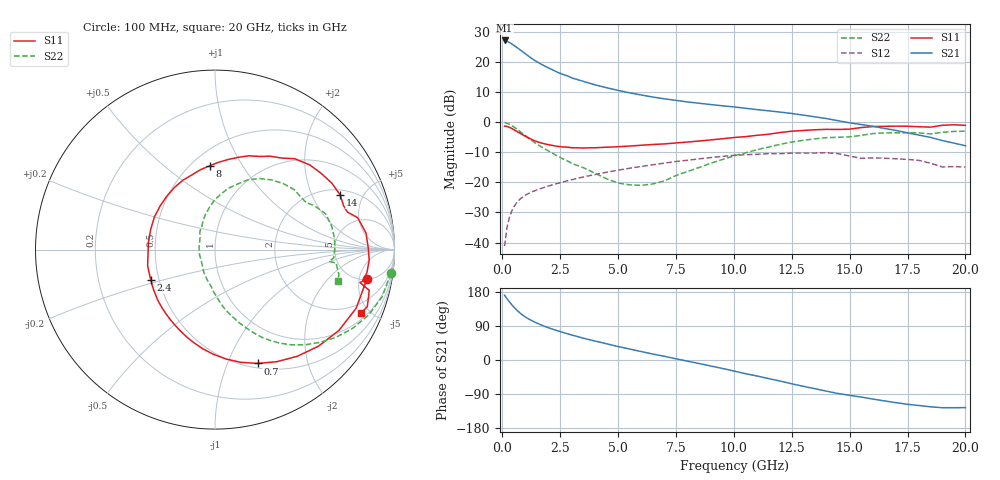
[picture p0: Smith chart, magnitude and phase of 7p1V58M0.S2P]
! Infineon Technologies  Discrete & RF Semiconductors
! bfp620
! VCE =  1.5 V,  IC =  8.0 mA
! Common Emitter S-Parameters:  Sep 2002
# GHz  S  MA  R  50
!  f  S11  S21  S12  S22
! GHz  MAG  ANG  MAG  ANG  MAG  ANG  MAG  ANG
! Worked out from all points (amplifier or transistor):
!   59 points, 100 MHz to 20 GHz, reference 50 ohm
!   highest |S21| = 27.2 dB at 100 MHz (marker M1)
!   |S21| within 3 dB of that: start of sweep to 747.6 MHz
!   unconditionally stable (mu >= 1): 4.357 GHz to 10.87 GHz; 17.09 GHz to end of sweep
!   at 1 GHz: K = 0.43, MSG = 23.5 dB, |S12| = -24.2 dB
!   at 5.5 GHz: K = 1.04, MAG = 11.2 dB, |S12| = -15.3 dB
!   at 20 GHz: K = 1.38, MAG = -0.1 dB, |S12| = -14.9 dB
!   S11 on the Smith chart (normalised r, x): 100 MHz: 5.18, -6.52; 700 MHz: 0.55, -1.29; 2.4 GHz: 0.45, -0.18; 8 GHz: 0.61, +0.73; 14 GHz: 2.28, +3.30; 20 GHz: 1.33, -4.40
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0.1  0.8621 -10.8  22.84 170.9  0.0087 84.8  0.9881 -7.6
0.2  0.8518 -22.5  22.2 162.0  0.0176 79.3  0.9676 -15.8
0.3  0.8245 -33.1  21.25 154.0  0.0256 73.8  0.9302 -23.1
0.4  0.7888 -43.0  20.13 146.5  0.0328 69.0  0.8835 -29.8
0.5  0.7505 -52.4  18.96 139.6  0.0392 64.8  0.8328 -35.9
0.6  0.7129 -61.2  17.81 133.3  0.0449 61.1  0.7813 -41.4
0.7  0.6772 -69.5  16.69 127.5  0.0498 58.0  0.731 -46.5
0.9  0.6124 -84.3  14.61 117.6  0.058 52.9  0.6375 -55.0
1  0.5832 -90.9  13.67 113.4  0.0614 50.9  0.5951 -58.5
1.2  0.532 -102.8  12 106.2  0.0673 47.7  0.5202 -64.4
1.4  0.4913 -113.4  10.65 100.1  0.0725 45.4  0.4583 -69.2
1.9  0.4309 -135.8  8.347 87.2  0.0846 41.6  0.3487 -79.1
2.4  0.3961 -154.5  6.728 76.9  0.0964 38.6  0.2717 -87.0
3.5  0.3734 173.8  4.769 57.6  0.1231 32.1  0.1756 -104.1
5  0.3911 140.9  3.378 35.5  0.1597 21.6  0.0975 -141.6
7  0.4356 107.1  2.446 9.8  0.2088 5.7  0.1056 142.2
8  0.468 93.6  2.169 -3.1  0.233 -3.7  0.1515 118.6
10.5  0.5757 64.3  1.704 -36.0  0.2882 -30.4  0.3098 84.2
13.5  0.749 29.6  1.228 -75.7  0.3086 -63.5  0.5291 44.1
14  0.761 23.6  1.15 -82.2  0.3106 -70.0  0.5541 37.0
17  0.861 -3.9  0.73 -112.7  0.2465 -94.4  0.6683 5.7
20  0.8865 -23.6  0.406 -125.6  0.1794 -106.6  0.7082 -14.5
